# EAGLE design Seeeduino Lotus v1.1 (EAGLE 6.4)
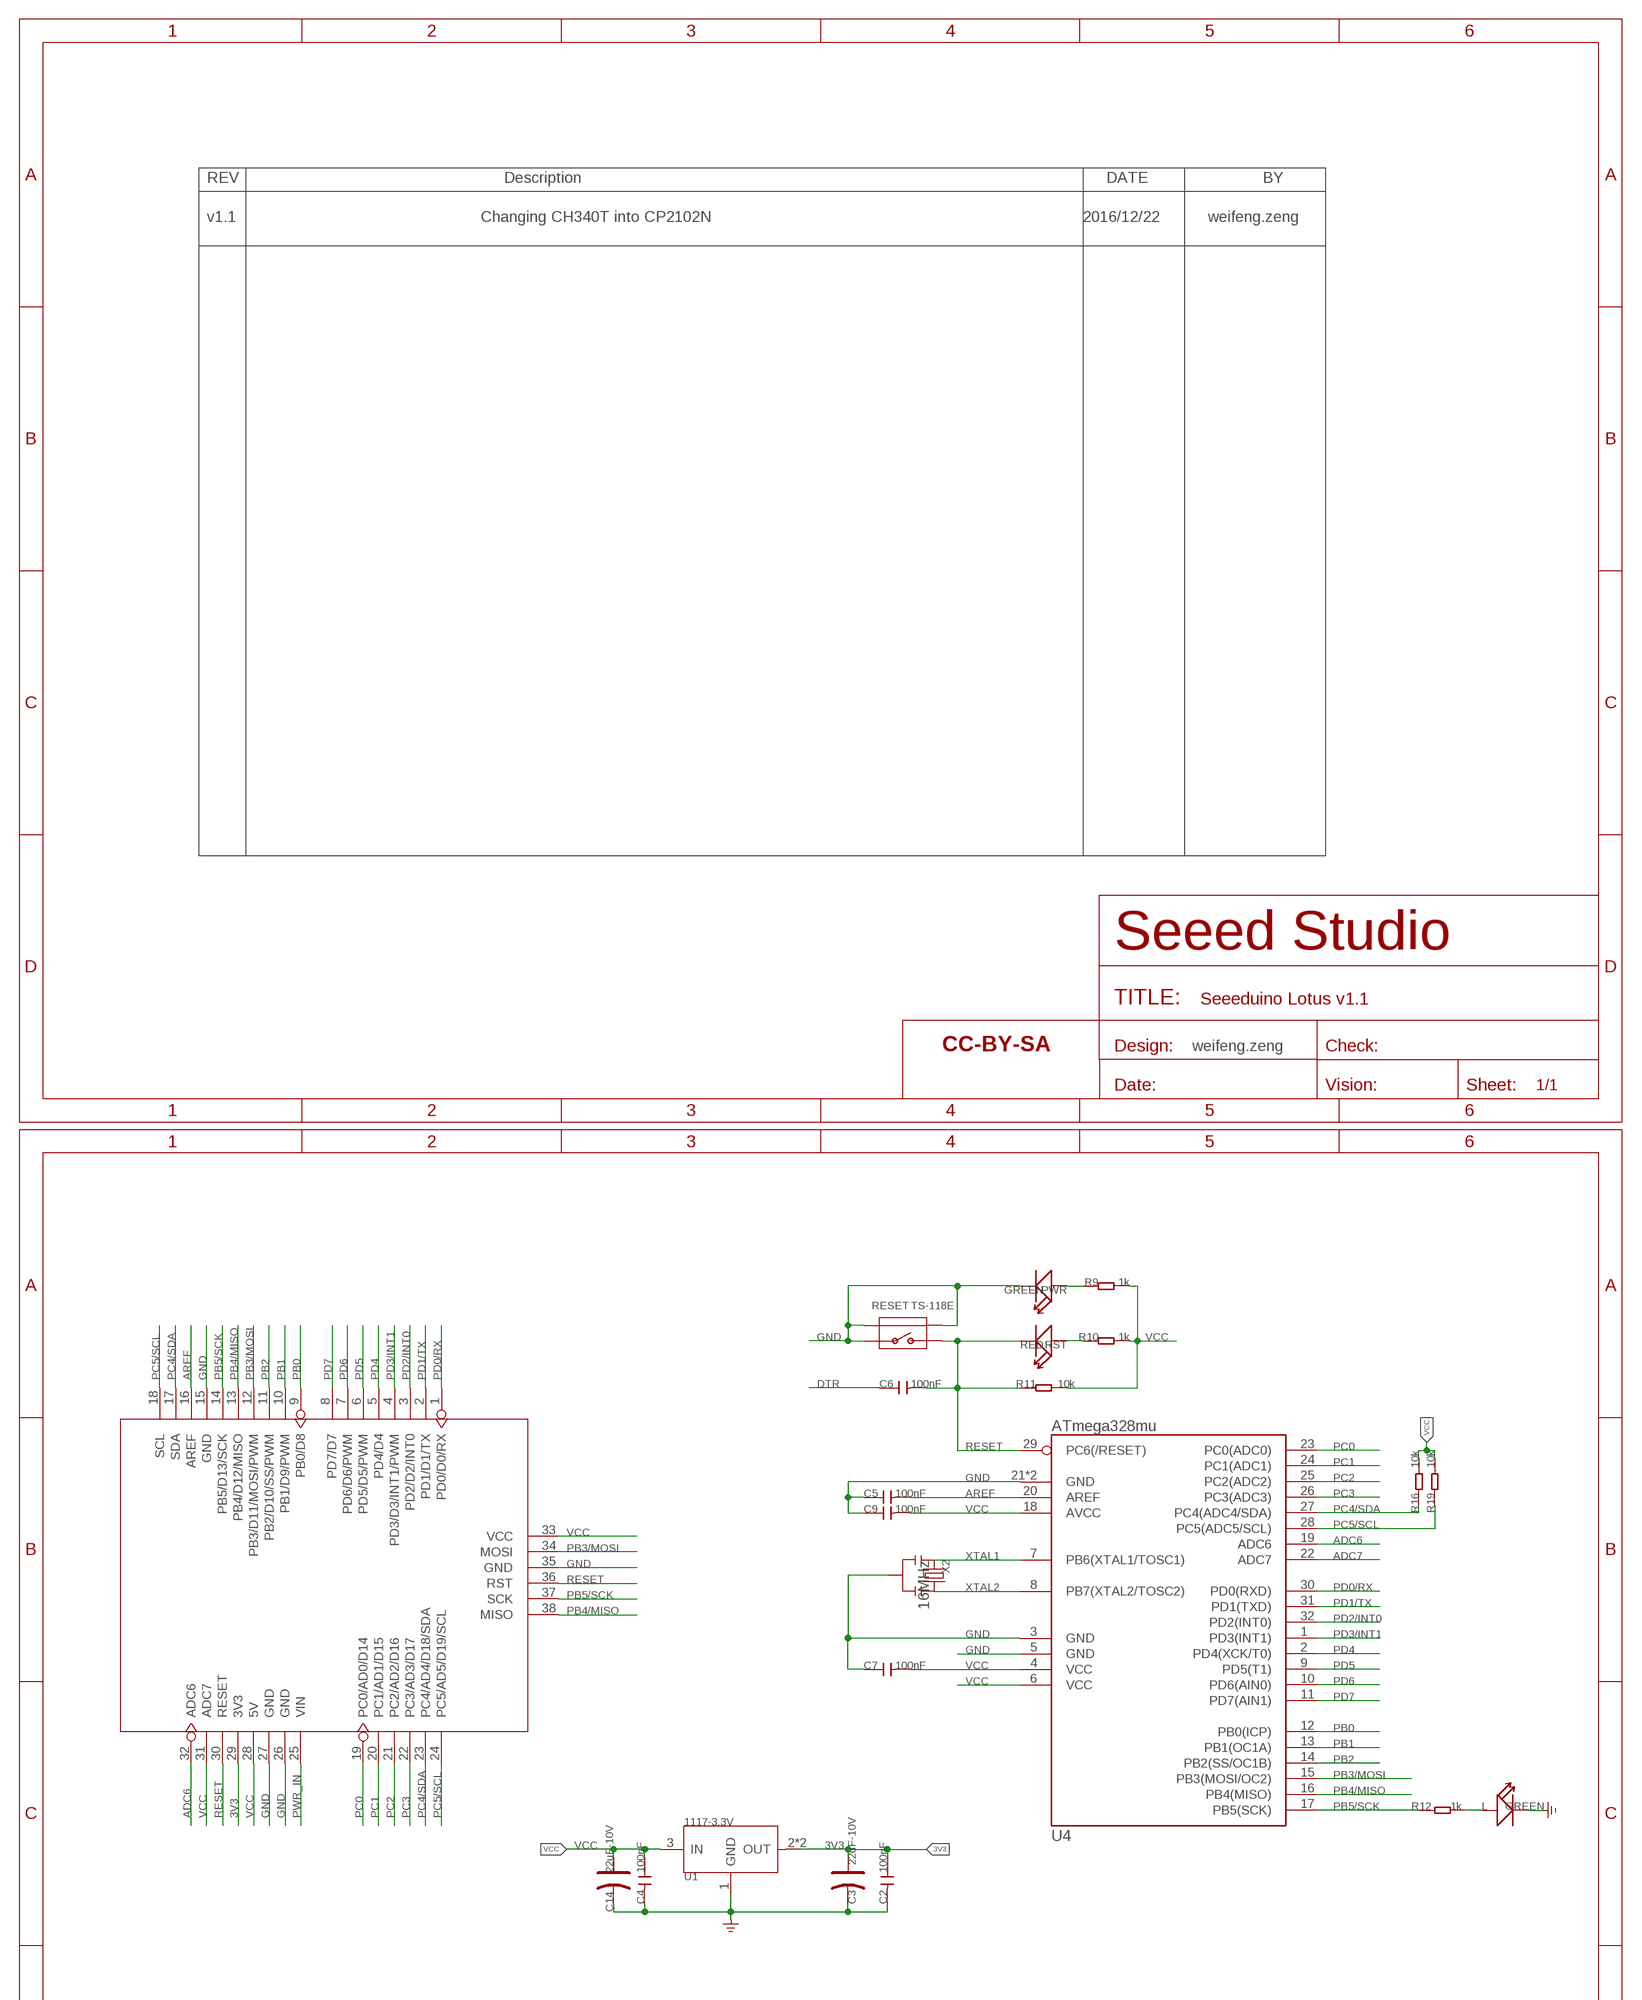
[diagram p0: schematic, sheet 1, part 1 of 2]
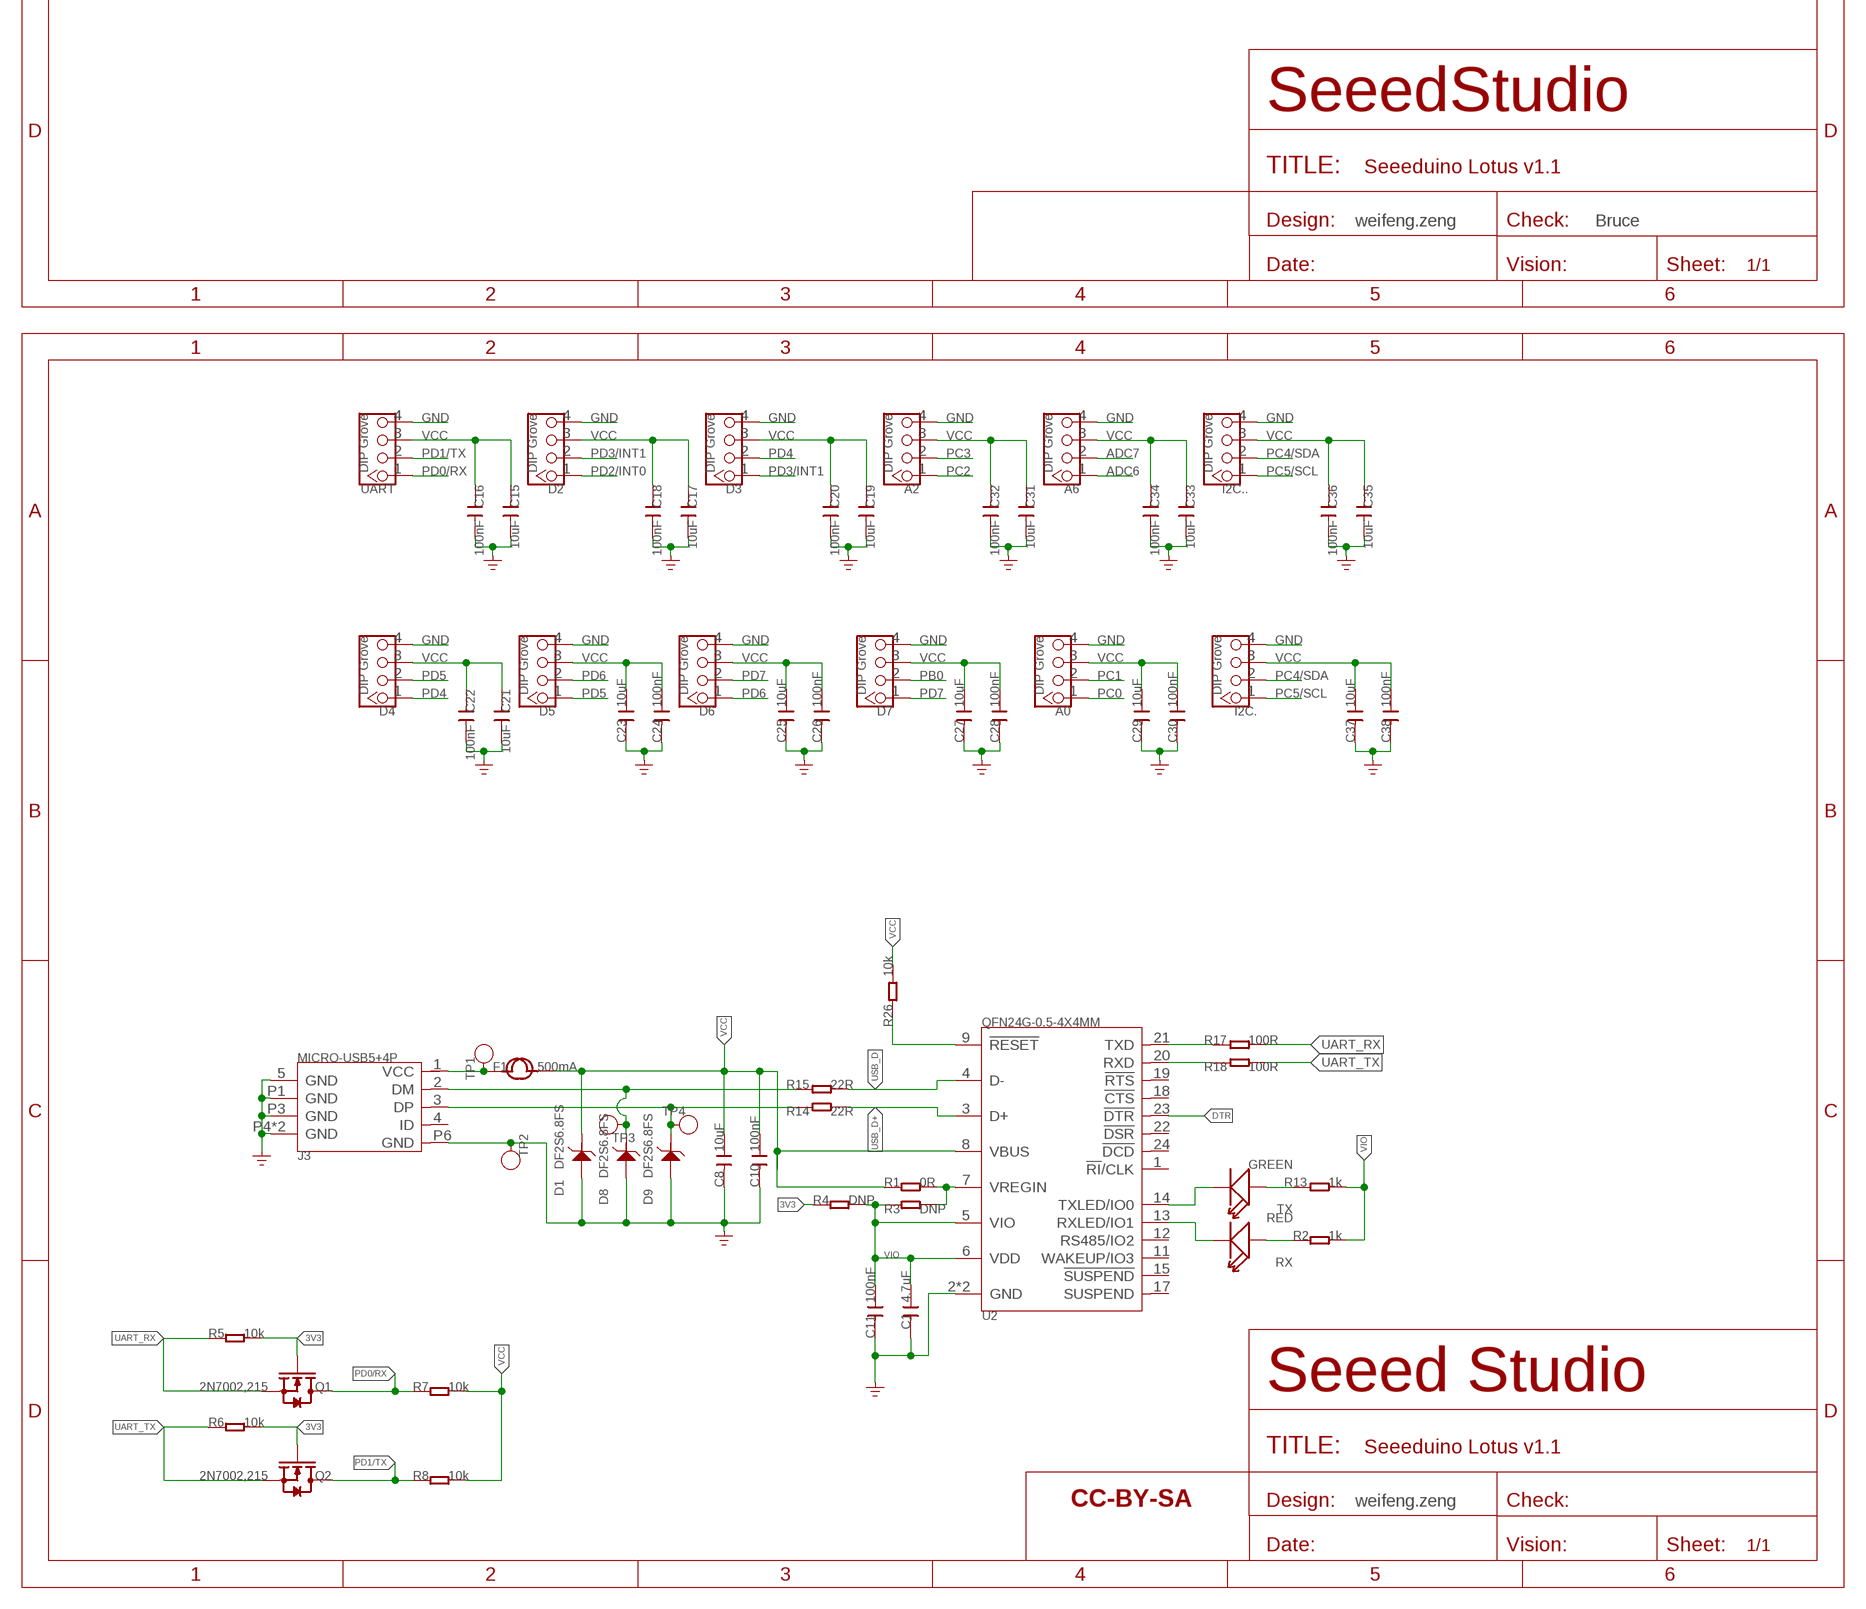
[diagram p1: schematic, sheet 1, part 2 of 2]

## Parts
A0  DIP Grove  TWIG-4P-2.0-2.0  [4P-2.0]
A2  DIP Grove  TWIG-4P-2.0-2.0  [4P-2.0]
A6  DIP Grove  TWIG-4P-2.0-2.0  [4P-2.0]
C1  4.7uF  CAP-0603  [C0603]
C2  100nF  CAP-0603  [C0603]
C3  22uF-10V  CAP-AVX-A  [AVX-A]
C4  100nF  CAP-0603  [C0603]
C5  100nF  CAP-0603  [C0603]
C6  100nF  CAP-0603  [C0603]
C7  100nF  CAP-0603  [C0603]
C8  10uF  CAP-0603  [C0603]
C9  100nF  CAP-0603  [C0603]
C10  100nF  CAP-0603  [C0603]
C11  100nF  CAP-0603  [C0603]
C14  22uF-10V  CAP-AVX-A  [AVX-A]
C15  10uF  CAP-0603  [C0603]
C16  100nF  CAP-0603  [C0603]
C17  10uF  CAP-0603  [C0603]
C18  100nF  CAP-0603  [C0603]
C19  10uF  CAP-0603  [C0603]
C20  100nF  CAP-0603  [C0603]
C21  10uF  CAP-0603  [C0603]
C22  100nF  CAP-0603  [C0603]
C23  10uF  CAP-0603  [C0603]
C24  100nF  CAP-0603  [C0603]
C25  10uF  CAP-0603  [C0603]
C26  100nF  CAP-0603  [C0603]
C27  10uF  CAP-0603  [C0603]
C28  100nF  CAP-0603  [C0603]
C29  10uF  CAP-0603  [C0603]
C30  100nF  CAP-0603  [C0603]
C31  10uF  CAP-0603  [C0603]
C32  100nF  CAP-0603  [C0603]
C33  10uF  CAP-0603  [C0603]
C34  100nF  CAP-0603  [C0603]
C35  10uF  CAP-0603  [C0603]
C36  100nF  CAP-0603  [C0603]
C37  10uF  CAP-0603  [C0603]
C38  100nF  CAP-0603  [C0603]
D1  DF2S6.8FS  D-ESD-2P'DF2S6.8FS'  [SOD-923]
D2  DIP Grove  TWIG-4P-2.0-2.0  [4P-2.0]
D3  DIP Grove  TWIG-4P-2.0-2.0  [4P-2.0]
D4  DIP Grove  TWIG-4P-2.0-2.0  [4P-2.0]
D5  DIP Grove  TWIG-4P-2.0-2.0  [4P-2.0]
D6  DIP Grove  TWIG-4P-2.0-2.0  [4P-2.0]
D7  DIP Grove  TWIG-4P-2.0-2.0  [4P-2.0]
D8  DF2S6.8FS  D-ESD-2P'DF2S6.8FS'  [SOD-923]
D9  DF2S6.8FS  D-ESD-2P'DF2S6.8FS'  [SOD-923]
F1  500mA  FUSE'1206'  [F1206]
FR1  SEEEDSTUDIO-OPEN-SCH-FRAME  [SEEEDSTUDIO-PCB-FRAME]
FR2  SEEEDSTUDIO-OPEN-SCH-FRAME  [SEEEDSTUDIO-PCB-FRAME]
I2C.  DIP Grove  TWIG-4P-2.0-2.0  [4P-2.0]
I2C..  DIP Grove  TWIG-4P-2.0-2.0  [4P-2.0]
J3  MICRO-USB5+4P  [MICRO-USB5+5P-SMD-0.65-7.2X5.06MM]
L  GREEN  LED'0603'  [LED-0603]
PWR  GREEN  LED'0603'  [LED-0603]
Q1  2N7002,215  MOSFET-N'SOT23'  [SOT-23]
Q2  2N7002,215  MOSFET-N'SOT23'  [SOT-23]
R1  0R  RES-0603  [R0603]
R2  1k  RES-0603  [R0603]
R3  DNP  RES-0603  [R0603]
R4  DNP  RES-0603  [R0603]
R5  10k  RES-0603  [R0603]
R6  10k  RES-0603  [R0603]
R7  10k  RES-0603  [R0603]
R8  10k  RES-0603  [R0603]
R9  1k  RES-0603  [R0603]
R10  1k  RES-0603  [R0603]
R11  10k  RES-0603  [R0603]
R12  1k  RES-0603  [R0603]
R13  1k  RES-0603  [R0603]
R14  22R  RES-0603  [R0603]
R15  22R  RES-0603  [R0603]
R16  10k  RES-0603  [R0603]
R17  100R  RES-0603  [R0603]
R18  100R  RES-0603  [R0603]
R19  10k  RES-0603  [R0603]
R26  10k  RES-0603  [R0603]
RESET  TS-118E  BUTTON-4P-REINFORCE'TS-1188E'  [4P-SMD-7X3.5X3.5H]
RST  RED  LED'0603'  [LED-0603]
RX  RED  LED'0603'  [LED-0603]
TP1  TEST-POINT'4545'  [TP-D45MIL]
TP2  TEST-POINT'4545'  [TP-D45MIL]
TP3  TEST-POINT'4545'  [TP-D45MIL]
TP4  TEST-POINT'4545'  [TP-D45MIL]
TX  GREEN  LED'0603'  [LED-0603]
U1  1117-3.3V  LD1117'SOT89'  [SOT89]
U2  QFN24G-0.5-4X4MM  CONVERTER-CP2102N(QFN24)  [QFN24G-0.5-4X4MM]
U3  ARDUINO-38P  [ARDUINO-38P]
U4  ATmega328mu  ATMEGA8/168/328MLF  [MLF32X-W/HEAT]
UART  DIP Grove  TWIG-4P-2.0-2.0  [4P-2.0]
X2  16MHz  CRYSTAL-RESONATOR'SMD'  [RESONATOR3-SMD-3.6X1.3X0.8MM]

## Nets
3V3: C2.1 C3.+ Q1.1(G) Q2.1(G) R4.1 R5.2 R6.2 U1.2(OUT) U1.4(OUT) U3.29(3V3)
ADC6: A6.1 U3.32(ADC6) U4.19(ADC6)
ADC7: A6.2 U4.22(ADC7)
AREF: C5.2 U3.16(AREF) U4.20(AREF)
D-: D8.1 J3.2(DM) R15.1 TP3.T
DTR: C6.1 U2.23(!DTR!)
GND: A0.4 A2.4 A6.4 C1.2 C2.2 C3.- C4.2 C5.1 C7.1 C8.2 C9.1 C10.2 C11.2 C14.- C15.1 C16.1 C17.1 C18.1 C19.1 C20.1 C21.1 C22.1 C23.2 C24.2 C25.2 C26.2 C27.2 C28.2 C29.2 C30.2 C31.1 C32.1 C33.1 C34.1 C35.1 C36.1 C37.2 C38.2 D1.2 D2.4 D3.4 D4.4 D5.4 D6.4 D7.4 D8.2 D9.2 I2C..4 I2C...4 J3.5(GND) J3.P1(GND) J3.P3(GND) J3.P4(GND) J3.P5(GND) J3.P6(GND) L.- PWR.- RESET.1 RESET.S1 RESET.S2 TP2.T U1.1(GND) U2.2(GND) U2.PAD(GND) U3.15(GND) U3.26(GND) U3.27(GND) U3.35(GND) U4.3(GND) U4.5(GND) U4.21(GND) U4.HEAT(GND) UART.4 X2.2 ; supply symbol labelled GND_POWER
N$1: R1.2 R3.2 U2.7(VREGIN)
N$2: R10.2 RST.+
N$3: PWR.+ R9.2
N$4: R26.2 U2.9(!RESET!)
N$5: TX.- U2.14(TXLED/IO0)
N$7: F1.1 J3.1(VCC) TP1.T
N$10: RX.- U2.13(RXLED/IO1)
N$11: D9.1 J3.3(DP) R14.1 TP4.T
N$13: L.+ R12.2
N$17: R18.1 U2.20(RXD)
N$18: R17.1 U2.21(TXD)
N$36: R2.1 RX.+
N$37: R13.1 TX.+
PB0: D7.2 U3.9(PB0/D8) U4.12(PB0(ICP))
PB1: U3.10(PB1/D9/PWM) U4.13(PB1(OC1A))
PB2: U3.11(PB2/D10/SS/PWM) U4.14(PB2(SS/OC1B))
PB3/MOSI: U3.12(PB3/D11/MOSI/PWM) U3.34(MOSI) U4.15(PB3(MOSI/OC2))
PB4/MISO: U3.13(PB4/D12/MISO) U3.38(MISO) U4.16(PB4(MISO))
PB5/SCK: R12.1 U3.14(PB5/D13/SCK) U3.37(SCK) U4.17(PB5(SCK))
PC0: A0.1 U3.19(PC0/AD0/D14) U4.23(PC0(ADC0))
PC1: A0.2 U3.20(PC1/AD1/D15) U4.24(PC1(ADC1))
PC2: A2.1 U3.21(PC2/AD2/D16) U4.25(PC2(ADC2))
PC3: A2.2 U3.22(PC3/AD3/D17) U4.26(PC3(ADC3))
PC4/SDA: I2C..2 I2C...2 R16.2 U3.17(SDA) U3.23(PC4/AD4/D18/SDA) U4.27(PC4(ADC4/SDA))
PC5/SCL: I2C..1 I2C...1 R19.2 U3.18(SCL) U3.24(PC5/AD5/D19/SCL) U4.28(PC5(ADC5/SCL))
PD0/RX: Q1.3(D) R7.1 U3.1(PD0/D0/RX) U4.30(PD0(RXD)) UART.1
PD1/TX: Q2.3(D) R8.1 U3.2(PD1/D1/TX) U4.31(PD1(TXD)) UART.2
PD2/INT0: D2.1 U3.3(PD2/D2/INT0) U4.32(PD2(INT0))
PD3/INT1: D2.2 D3.1 U3.4(PD3/D3/INT1/PWM) U4.1(PD3(INT1))
PD4: D3.2 D4.1 U3.5(PD4/D4) U4.2(PD4(XCK/T0))
PD5: D4.2 D5.1 U3.6(PD5/D5/PWM) U4.9(PD5(T1))
PD6: D5.2 D6.1 U3.7(PD6/D6/PWM) U4.10(PD6(AIN0))
PD7: D6.2 D7.1 U3.8(PD7/D7) U4.11(PD7(AIN1))
PWR_IN: U3.25(VIN)
RESET: C6.2 R11.2 RESET.2 RST.- U3.30(RESET) U3.36(RST) U4.29(PC6(/RESET))
UART_RX: Q1.2(S) R5.1 R17.2
UART_TX: Q2.2(S) R6.1 R18.2
USB_D: R15.2 U2.4(D-)
USB_D+: R14.2 U2.3(D+)
VCC: A0.3 A2.3 A6.3 C4.1 C7.2 C8.1 C9.2 C10.1 C14.+ C15.2 C16.2 C17.2 C18.2 C19.2 C20.2 C21.2 C22.2 C23.1 C24.1 C25.1 C26.1 C27.1 C28.1 C29.1 C30.1 C31.2 C32.2 C33.2 C34.2 C35.2 C36.2 C37.1 C38.1 D1.1 D2.3 D3.3 D4.3 D5.3 D6.3 D7.3 F1.2 I2C..3 I2C...3 R1.1 R7.2 R8.2 R9.1 R10.1 R11.1 R16.1 R19.1 R26.1 U1.3(IN) U2.8(VBUS) U3.28(5V) U3.31(ADC7) U3.33(VCC) U4.4(VCC) U4.6(VCC) U4.18(AVCC) UART.3
VIO: C1.1 C11.1 R2.2 R3.1 R4.2 R13.2 U2.5(VIO) U2.6(VDD)
XTAL1: U4.7(PB6(XTAL1/TOSC1)) X2.1
XTAL2: U4.8(PB7(XTAL2/TOSC2)) X2.3
Unconnected: J3.4(ID) U2.1(!RI!/CLK) U2.11(WAKEUP/IO3) U2.12(RS485/IO2) U2.15(!SUSPEND!) U2.17(SUSPEND) U2.18(!CTS!) U2.19(!RTS!) U2.22(!DSR!) U2.24(!DCD!)

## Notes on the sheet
- v1.1 | Changing CH340T into CP2102N | 2016/12/22 | weifeng.zeng
- weifeng.zeng
- weifeng.zeng | Bruce
- weifeng.zeng

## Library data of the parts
A0 A2 A6 = Connector :TWIG-4P-2.0
C1 C2 C4 C8 C10 C11 C15-C38 = Discrete-new:CAP: Ceramic Capacitors
C3 C14 = Discrete:CAP*: Electrolytic Capacitors,Tantalum Capacitors and Super Capacitors
C5-C7 C9 = C-R-package test:CAP: Ceramic Capacitors
D1 D8 D9 = Discrete-new:D-ESD-2P: SOD-923:304060009;SOD-123:304060001
D2-D7 I2C. I2C.. UART = Connector:TWIG-4P-2.0
F1 = Discrete-new:FUSE
FR1 FR2 = moudle-new:SEEEDSTUDIO-OPEN-SCH-FRAME
J3 = Connector-new:MICRO-USB5+4P: 5+4P-SMD-0.65-B:320010000;5+2P-SMD-0.65-AB:340032001;5+5P-SMD-0.65-7.2X5.06MM:320010050;
L PWR RST = Discrete:LED*
Q1 Q2 = Discrete-new:MOSFET-N
R1-R8 R13-R19 R26 = Discrete-new:RES
R9-R12 = C-R-package test:RES
RESET = Discrete:BUTTON-4P-REINFORCE: TS-1188E http://www.best-dz.com/?thread-374-2.html
RX TX = Discrete-new:LED
TP1-TP4 = Discrete-new:TEST-POINT; PARTNO: DNP
U1 = IC:LD1117: Low Drop Fixed And Adjustable Positive Voltage Regulators http://www.datasheetcatalog.org/datasheet/SGSThomsonMicroelectronics/mXuqtqv.pdf
U2 = template:CONVERTER-CP2102N(QFN24)
U3 = moudle:ARDUINO-38P
U4 = IC:ATMEGA8/168/328: MICROCONTROLLER
X2 = Discrete-new:CRYSTAL-RESONATOR: Resonator Small SMD resonator. This is the itty bitty 10/20MHz resonators with built in caps. CSTCE10M0G55 and CSTCE20M0V53. Footprint has been reviewed closely but hasn't been tested yet.

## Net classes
3 usbvcc: width 0.203 mm, drill 0.305 mm, clearance 0.203 mm

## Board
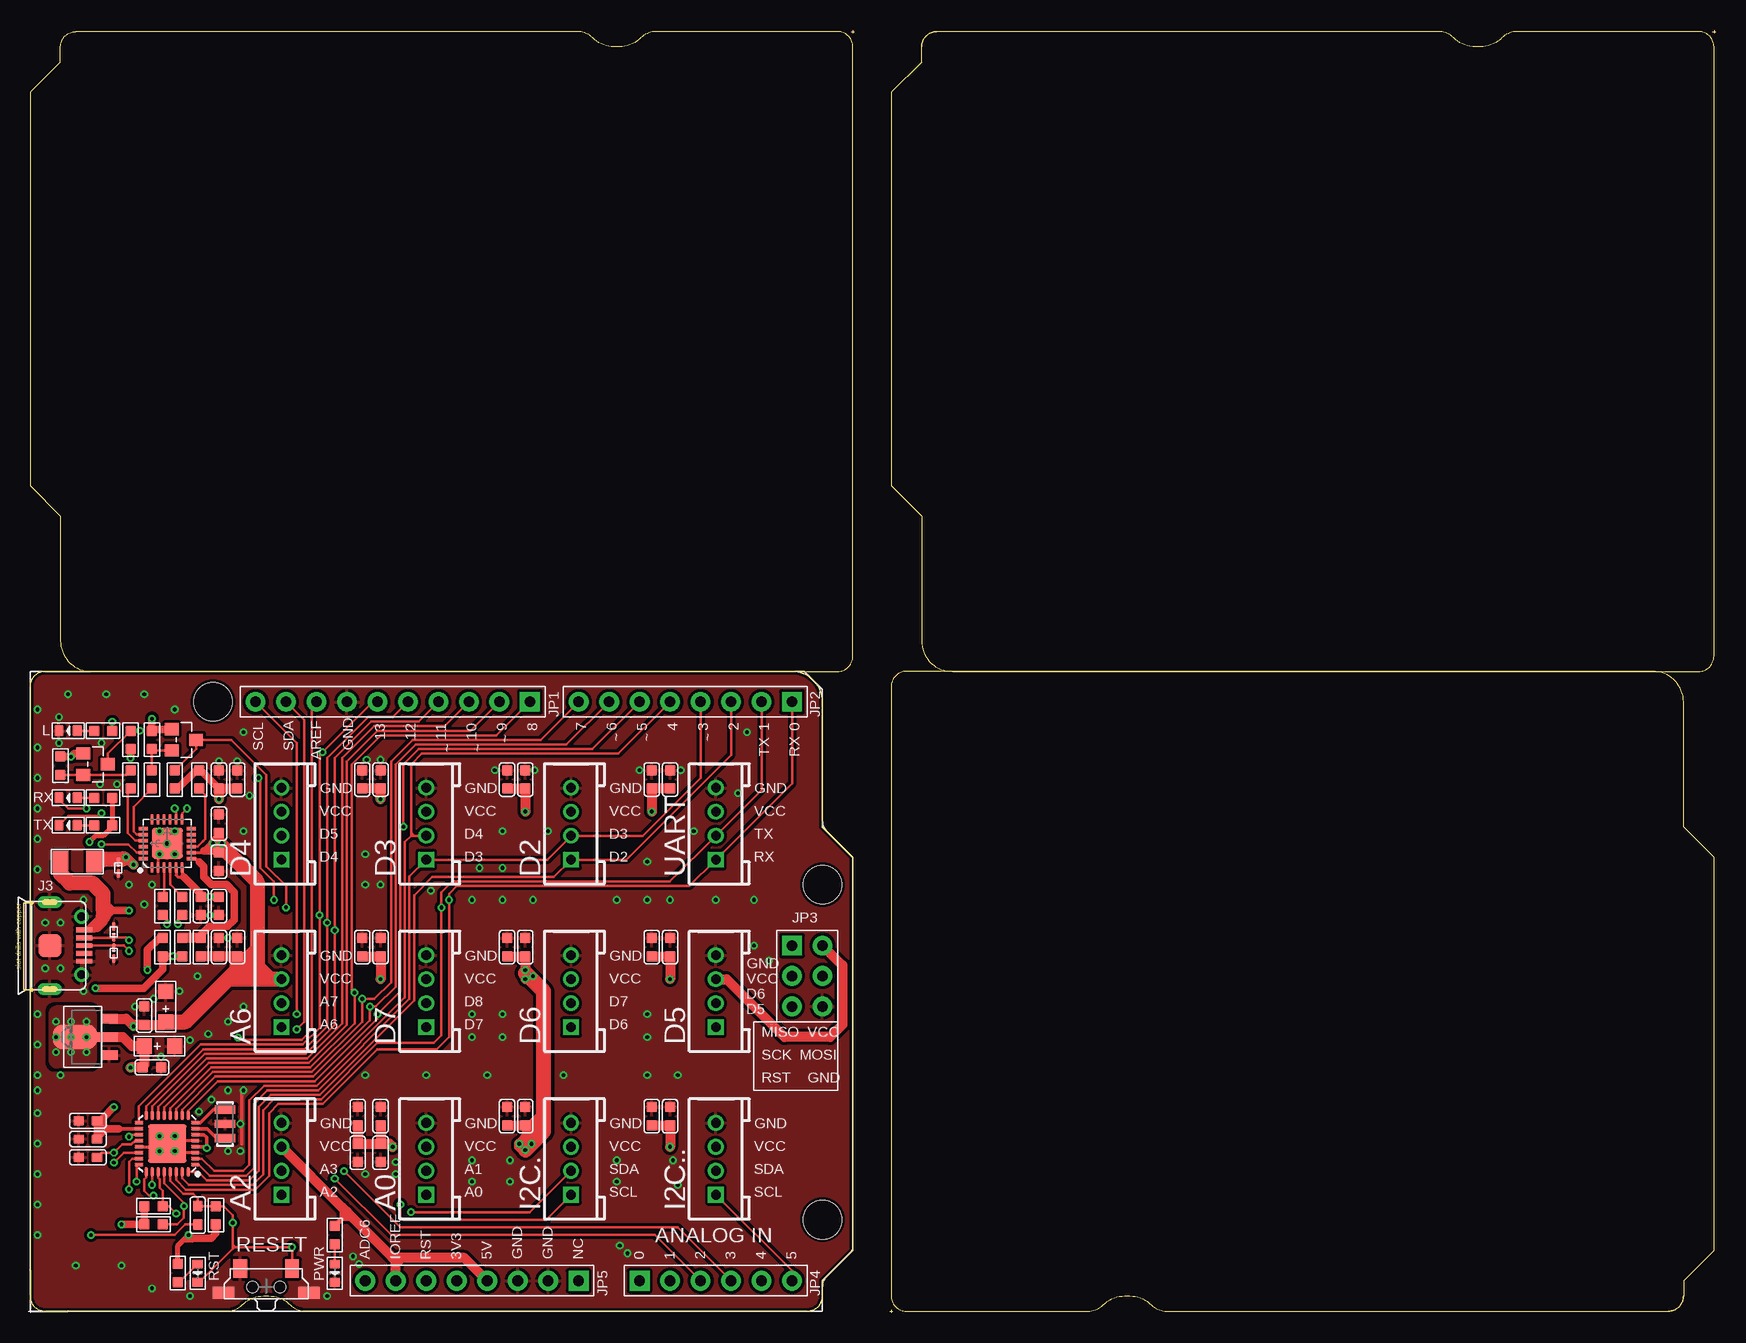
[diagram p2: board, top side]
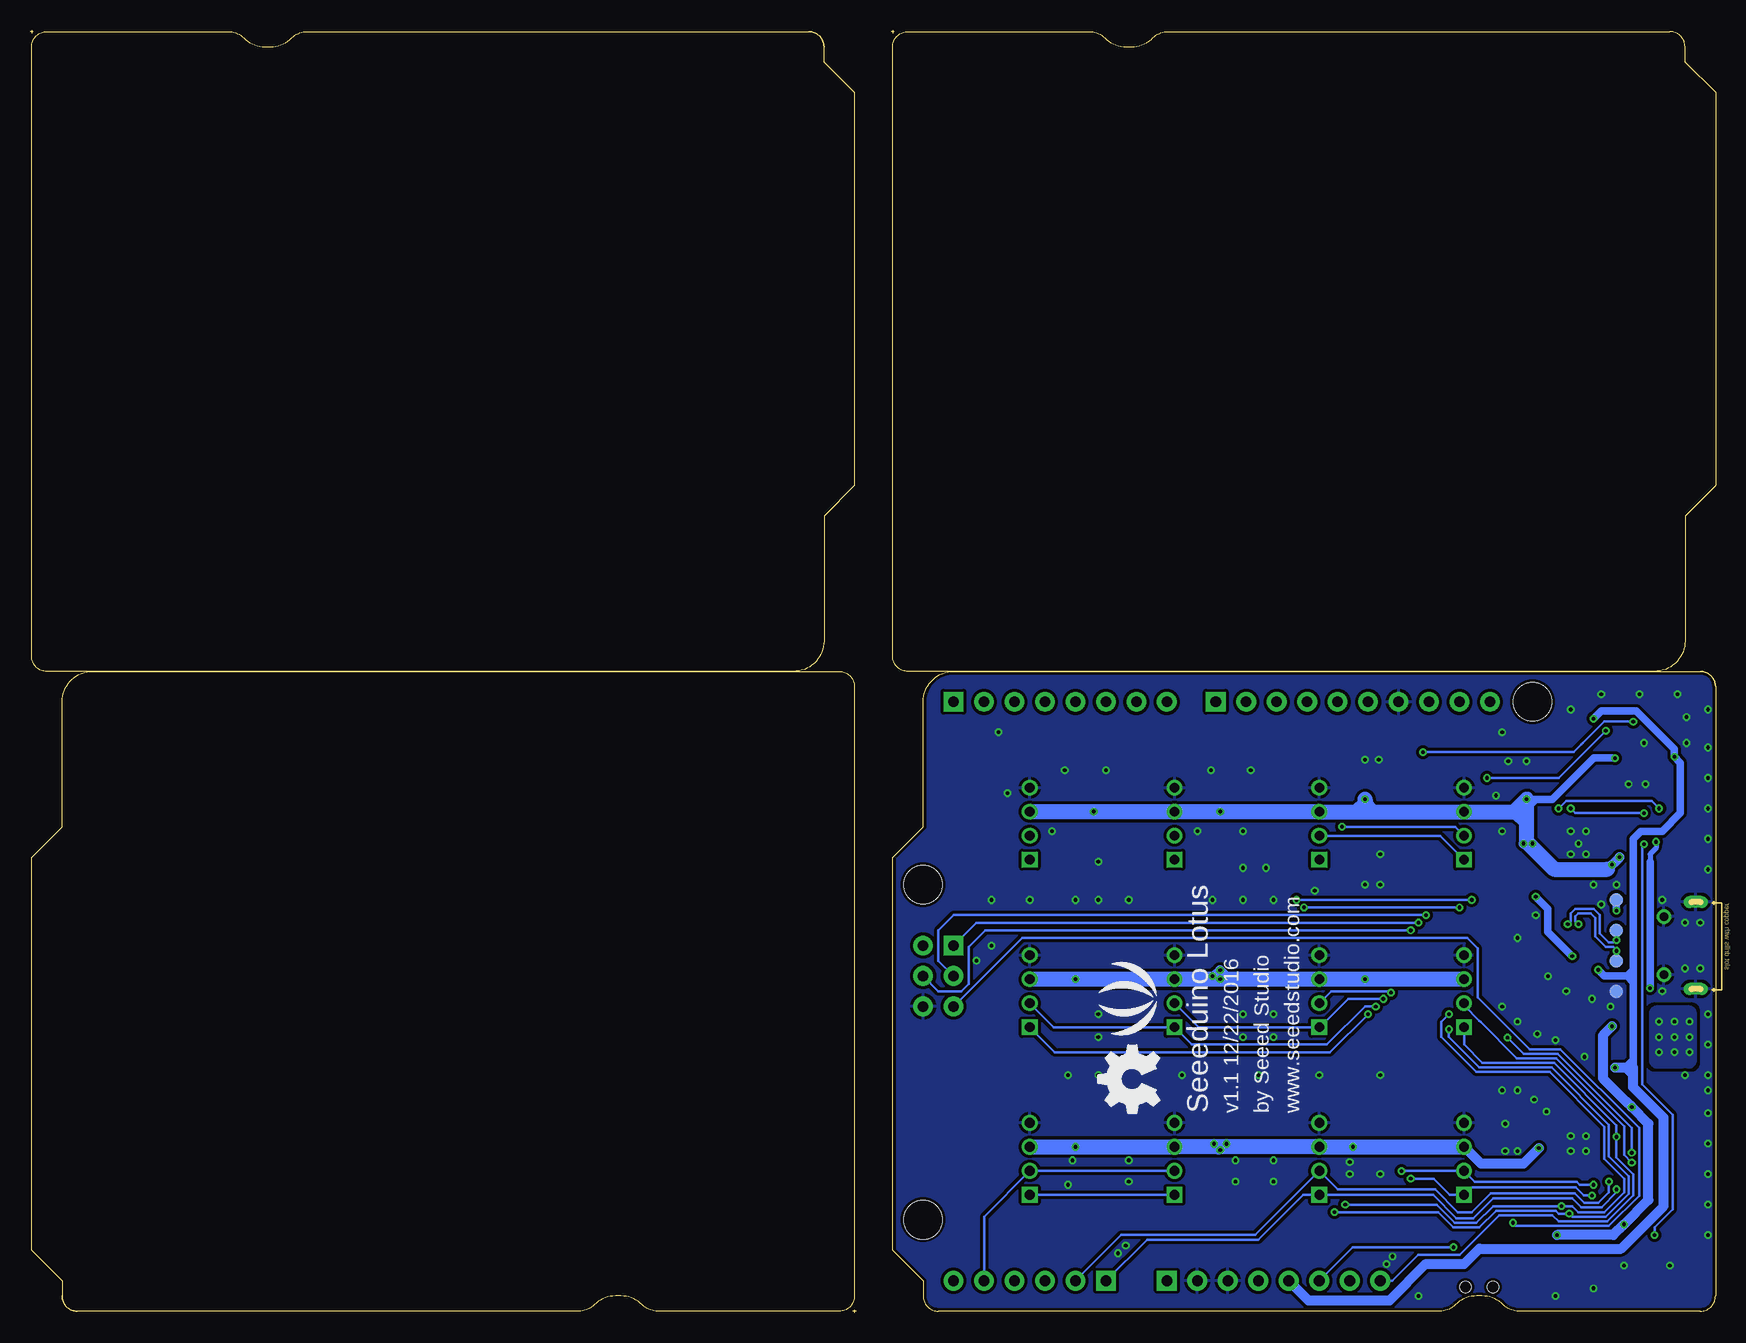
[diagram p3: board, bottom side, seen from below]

Size 140.46 x 106.93 mm. Coordinates in mm from the lower left corner, seen from the top.
Outline: 125 segments
Copper layers (1*16): Top 0.035mm / dielectric 1.5mm / Bottom 0.035mm
Design rules "SeeedStudio_rule_no_angle_090911 *": minimum track width 1mil, minimum drill 12mil, track to track 6mil, track to pad 6mil, pad to pad 6mil, via to via 6mil, smd to smd 0mil, copper to edge 10mil, drill to drill 10mil, minimum pad ring 10mil, minimum via ring 6mil, stop-mask expansion 2mil, vias tented up to drill 100mil, thermal gap 10mil
Holes 2.03 mm at 7.62,111.25 132.72,111.25 132.72,-4.32 7.62,-4.32

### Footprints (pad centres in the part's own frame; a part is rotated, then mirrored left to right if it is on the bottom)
4P-2.0 = drill 0.8 pad 1.27 square: 1 -3,0 | drill 0.8 pad 1.27: 2 -1,0; 3 1,0; 4 3,0
C0603 = smd 0.889 x 0.889: 1 0,0.762; 2 0,-0.762
AVX-A = smd 1.27 x 1.27: + -1.27,0; - 1.27,0
C0603' = smd 0.762 x 0.889: 1 0,0.762; 2 0,-0.762
SOD-923 = smd 0.7 x 0.3: 1 -0.45,0; 2 0.45,0
F1206 = smd 1.27 x 1.778: 1 -1.397,0; 2 1.397,0
MICRO-USB5+5P-SMD-0.65-7.2X5.06MM = smd 0.4 x 1.35: 1 -1.3,2.875; 2 -0.65,2.875; 3 0,2.875; 4 0.65,2.875; 5 1.3,2.875 | smd 1.9 x 1.9: P1 0,0 | drill 0.508 pad 1.016 long: P3 -3.625,0; P4 3.625,0 | drill 0.7: P5 -2.425,2.65; P6 2.425,2.65
LED-0603 = smd 0.762 x 0.889: + -0.762,0; - 0.762,0
SOT-23 = smd 1.016 x 1.143: 1 -0.889,-1.016; 2 0.889,-1.016; 3 0,1.016
R0603 = smd 0.889 x 0.889: 1 0,0.762; 2 0,-0.762
4P-SMD-7X3.5X3.5H = smd 1.143 x 1.524: 1 -2.159,1.524; 2 2.159,1.524 | smd 1.778 x 1.016: S1 -3.556,-0.508; S2 3.556,-0.508 | hole 0.95: -1.15,0; 1.15,0
TP-D45MIL = smd 1.143 x 1.143: T 0,0
SOT89 = smd 0.8 x 1.4: 1 -1.524,-1.905; 3 1.524,-1.905 | smd 0.8 x 1.9: 2 0,-1.651 | smd 2.032 x 3.65: 4 0,0.94
QFN24G-0.5-4X4MM = smd 0.8 x 0.26: 1 -2,1.25; 2 -2,0.75; 3 -2,0.25; 4 -2,-0.25; 5 -2,-0.75; 6 -2,-1.25; 13 2,-1.25; 14 2,-0.75; 15 2,-0.25; 16 2,0.25; 17 2,0.75; 18 2,1.25 | smd 0.26 x 0.8: 7 -1.25,-2; 8 -0.75,-2; 9 -0.25,-2; 10 0.25,-2; 11 0.75,-2; 12 1.25,-2; 19 1.25,2; 20 0.75,2; 21 0.25,2; 22 -0.25,2; 23 -0.75,2; 24 -1.25,2 | smd 2.6 x 2.6: PAD 0.02,-0.01
ARDUINO-38P = drill 0.889 pad 1.651 square: 1 63.5,50.8; 9 41.656,50.8; 19 50.8,2.54; 25 45.72,2.54; 38 63.5,30.48 | drill 0.889 pad 1.651: 2 60.96,50.8; 3 58.42,50.8; 4 55.88,50.8; 5 53.34,50.8; 6 50.8,50.8; 7 48.26,50.8; 8 45.72,50.8; 10 39.116,50.8; 11 36.576,50.8; 12 34.036,50.8; 13 31.496,50.8; 14 28.956,50.8; 15 26.416,50.8; 16 23.876,50.8; 17 21.336,50.8; 18 18.796,50.8; 20 53.34,2.54; 21 55.88,2.54; 22 58.42,2.54; 23 60.96,2.54; 24 63.5,2.54; 26 43.18,2.54; 27 40.64,2.54; 28 38.1,2.54; 29 35.56,2.54; 30 33.02,2.54; 31 30.48,2.54; 32 27.94,2.54; 33 66.04,30.48; 34 66.04,27.94; 35 66.04,25.4; 36 63.5,25.4; 37 63.5,27.94 | hole 3.2: 15.24,50.8; 66.04,35.56; 66.04,7.62
MLF32X-W/HEAT = smd 0.7 x 0.3: 1 -2.35,1.75; 2 -2.35,1.25; 3 -2.35,0.75; 4 -2.35,0.25; 5 -2.35,-0.25; 6 -2.35,-0.75; 7 -2.35,-1.25; 8 -2.35,-1.75; 17 2.35,-1.75; 18 2.35,-1.25; 19 2.35,-0.75; 20 2.35,-0.25; 21 2.35,0.25; 22 2.35,0.75; 23 2.35,1.25; 24 2.35,1.75 | smd 0.3 x 0.7: 9 -1.75,-2.35; 10 -1.25,-2.35; 11 -0.75,-2.35; 12 -0.25,-2.35; 13 0.25,-2.35; 14 0.75,-2.35; 15 1.25,-2.35; 16 1.75,-2.35; 25 1.75,2.35; 26 1.25,2.35; 27 0.75,2.35; 28 0.25,2.35; 29 -0.25,2.35; 30 -0.75,2.35; 31 -1.25,2.35; 32 -1.75,2.35 | smd 3.175 x 3.175: HEAT 0,0
RESONATOR3-SMD-3.6X1.3X0.8MM = smd 0.7 x 1.7: 1 -1.2,0; 2 0,0; 3 1.2,0

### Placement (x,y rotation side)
A0  33.02,12.83 90 top
A2  20.95,12.83 90 top
A6  20.95,26.8 90 top
C1  15.75,33.91 0 top
C2  10.16,20.45 90 top
C3  10.79,22.22 0 top
C4  9.53,24.77 180 top
C5  100nF  [C0603']  4.83,12.95 90 top
C6  100nF  [C0603']  13.97,8.13 180 top
C7  100nF  [C0603']  4.83,16 90 top
C8  15.75,37.59 0 top
C9  100nF  [C0603']  4.83,14.48 90 top
C10  15.75,40.77 180 top
C11  14.22,33.91 0 top
C14  11.3,25.53 90 top
C15  51.82,44.45 0 top
C16  53.34,44.45 0 top
C17  39.75,44.45 0 top
C18  41.27,44.45 0 top
C19  27.69,44.45 0 top
C20  29.21,44.45 0 top
C21  15.75,44.45 0 top
C22  17.27,44.45 0 top
C23  51.82,30.48 180 top
C24  53.34,30.48 180 top
C25  39.75,30.48 180 top
C26  41.27,30.48 180 top
C27  27.69,30.48 180 top
C28  29.21,30.48 180 top
C29  29.21,13.34 0 top
C30  29.21,16.38 180 top
C31  27.3,13.34 180 top
C32  27.3,16.38 0 top
C33  15.75,30.48 0 top
C34  17.27,30.48 0 top
C35  51.82,16.38 0 top
C36  53.34,16.38 0 top
C37  39.75,16.38 180 top
C38  41.27,16.38 180 top
D1  7.37,37.08 270 top
D2  45.09,40.77 90 top
D3  33.02,40.77 90 top
D4  20.95,40.77 90 top
D5  57.15,26.8 90 top
D6  45.09,26.8 90 top
D7  33.02,26.8 90 top
D8  6.99,31.75 90 top
D9  6.99,29.97 270 top
F1  3.94,37.59 0 top
FR1  not placed on the board
FR2  not placed on the board
I2C.  45.09,12.83 90 top
I2C..  57.15,12.83 90 top
J3  1.65,30.61 270 top
L  3.17,48.51 180 top
PWR  25.4,3.3 270 top
Q1  5.46,45.72 270 top
Q2  12.83,47.75 270 top
R1  14.22,30.48 180 top
R2  6.1,42.93 90 top
R3  12.7,30.48 180 top
R4  11.05,30.48 0 top
R5  2.54,45.59 180 top
R6  10.16,47.75 180 top
R7  8.38,47.75 0 top
R8  12.06,44.45 0 top
R9  25.4,6.48 0 top
R10  12.32,3.3 0 top
R11  15.49,8.13 180 top
R12  6.1,48.51 270 top
R13  6.1,40.64 90 top
R14  11.05,33.91 180 top
R15  12.7,33.91 180 top
R16  10.29,8.89 90 top
R17  8.38,44.45 180 top
R18  10.16,44.45 180 top
R19  10.29,7.37 90 top
R26  14.1,44.45 0 top
RESET  19.68,2.16 0 top
RST  13.97,3.3 270 top
RX  3.17,42.93 180 top
TP1  8.26,34.42 180 bottom
TP2  8.26,26.8 180 bottom
TP3  8.26,31.88 180 bottom
TP4  8.26,29.34 180 bottom
TX  3.17,40.64 180 top
U1  4.7,22.99 90 top
U2  11.43,39.12 90 top
U3  0,0.13 0 top
U4  11.43,14.1 180 top
U$2  [OSHW_FILLX200_NOTEXT]  46.35,16.64 90 bottom
U$4  [LOGO_SILK]  48.26,26.16 90 bottom
U$12  [SEEED_MASK]  3.81,2.67 0 top
UART  57.15,40.77 90 top
X2  16.26,15.75 90 top

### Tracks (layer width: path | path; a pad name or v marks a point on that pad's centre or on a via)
3V3  (via drill 0.3 pad 0.64)
  Top 0.61: v4.7,22.99 U1.4 | 9.53,20.57 C2.1 | R4.1 10.79,31.24 9.78,30.23 v9.78,28.57 | R5.2 v3.43,46.36 3.68,46.61 Q1.1 | Q2.1 10.29,48.64 R6.2 v10.16,49.53
  Top 0.813: C2.1 9.27,20.45 | 9.27,20.45 v8.38,20.45 | 9.27,20.45 9.53,20.7 C3.+ 8.51,22.22 7.75,22.99 U1.2
  Bottom 0.61: 6.86,20.45 6.86,21.08 | 6.86,21.08 6.86,27.56 | 6.86,27.56 6.86,28.07 | 6.86,28.07 6.86,28.57 | 7.37,28.07 6.86,28.07 | 7.37,28.07 6.86,28.57 | 7.37,28.07 6.86,27.56 | 7.37,28.07 9.27,28.07 v9.78,28.57 | 6.86,28.57 6.86,39.5 6.22,40.13 4.45,40.13 2.92,41.66 2.92,45.85 v3.43,46.36 3.43,46.99 6.6,50.16 9.53,50.16 v10.16,49.53 | 6.86,21.08 7.49,20.45 | 7.75,20.45 7.62,20.45 6.86,19.68
  Bottom 0.813: U3.29 33.91,1.02 27.18,1.02 24.13,4.06 20.95,4.06 19.68,5.33 7.87,5.33 4.32,8.89 4.32,16.26 6.86,18.8 6.86,19.68 6.86,20.45 7.49,20.45 7.75,20.45 v8.38,20.45
  other vias: 4.7,24.26 3.43,24.26 2.16,24.26 3.43,22.99 2.16,22.99 2.16,21.72 3.43,21.72 4.7,21.72
  pour Top (isolate 0.254, no thermals): 4.83,20.45 2.29,20.45 arc-90 1.65,21.08 1.65,24.89 arc-90 2.29,25.53 4.83,25.53 arc-90 5.46,24.89 5.46,21.08 arc-90
  pour Bottom (isolate 0.254, no thermals): 4.83,20.45 2.29,20.45 arc-90 1.65,21.08 1.65,24.89 arc-90 2.29,25.53 4.83,25.53 arc-90 5.46,24.89 5.46,21.08 arc-90
ADC6  (via drill 0.3 pad 0.64)
  Top 0.203: U4.19 8.43,14.85 v8.26,14.67
  Bottom 0.203: U3.32 26.92,2.67 24.77,4.83 21.34,4.83 18.03,8.13 13.59,8.13 13.08,7.62 9.02,7.62 6.86,9.78 6.86,11.56 8.26,12.95 v8.26,14.67 8.26,15.63 13.46,20.83 19.43,20.83 20.95,22.35 A6.1
ADC7  (via drill 0.3 pad 0.64)
  Top 0.203: U4.22 7.82,13.35 v6.99,12.51
  Bottom 0.203: v6.99,12.51 7.62,13.15 7.62,15.54 13.28,21.21 16.56,21.21 19.58,24.23 19.68,24.33 20.95,25.6 A6.2
AREF  (via drill 0.3 pad 0.64)
  Top 0.203: U3.16 23.5,50.55 23.5,23.62 22.63,22.75 17.51,22.75 v17.34,22.92 | U4.20 8.76,14.35 8.45,14.03 7.68,14.03 v6.99,13.34 5.97,13.34 C5.2
  Bottom 0.203: v6.99,13.34 6.99,15.43 13.14,21.59 16,21.59 v17.34,22.92
D-  (via drill 0.3 pad 0.64)
  Top 0.203: J3.2 6.94,31.26 D8.1 8.01,31.3 v8.26,31.05 | R15.1 12.32,32.77 v12.32,32.39
  Bottom 0.203: TP3.T v8.26,31.05 8.32,31.05 8.51,30.86 8.89,30.86 9.65,31.62 9.65,33.15 10.16,33.66 11.68,33.66 12.06,33.27 12.06,32.64 v12.32,32.39
DTR  (via drill 0.3 pad 0.64)
  Top 0.203: C6.1 12.95,7.37 12.06,6.48 v5.08,6.48 | U2.23 8.88,38.37 8.19,39.05 v5.97,39.05
  Bottom 0.203: v5.97,39.05 6.1,38.93 6.1,19.05 3.56,16.51 3.56,8.64 5.08,7.11 v5.08,6.48
GND  (via drill 0.3 pad 0.64)
  Top 0.203: U2.2 10.68,38.11 v10.79,38.23
  Top 0.254: U4.21 9.91,13.85 v10.79,14.73 U4.HEAT | U4.3 12.18,13.35 v12.06,13.46 | U4.5 12.45,14.35 v12.06,14.73
  Top 0.305: 17.65,14.1 17.65,18.54
  other vias: 36.83,24.89 39.37,24.89 39.37,22.99 36.83,22.99 51.44,24.89 51.44,22.99 48.9,12.7 40.01,10.92 53.59,12.7 48.9,10.92 40.01,12.7 53.98,10.67 30.48,12.57 26.92,4.7 27.43,4.06 60.33,30.61 61.59,29.34 37.47,37.08 39.37,37.08 49.15,5.59 49.78,4.95 30.48,11.56 36.83,10.92 36.83,12.7 10.79,13.46 0.64,19.81 2.54,19.81 0.64,18.54 0.64,6.48 7.62,3.94 17.78,18.54 17.53,15.75 16.51,13.46 17.53,13.46 27.94,11.56 27.94,19.81 33.02,19.81 38.1,19.81 44.45,19.81 51.44,19.81 53.98,19.81 36.83,34.42 39.37,34.42 41.91,34.42 43.18,40.13 39.37,40.13 51.44,37.59 48.9,34.42 51.44,34.42 53.34,34.42 60.33,34.42 57.15,34.42 3.81,3.94 14.99,33.15 16.51,31.24 29.21,46.1 28.07,46.1 29.21,35.69 27.94,35.69 11.43,39.12 12.06,40.13 10.79,40.13 12.06,38.23 8.26,35.69 10.16,35.69 9.53,34.04 17.78,40.13 0.64,11.56 0.64,16.64 0.64,14.1 0.64,9.02 0.64,22.35 0.64,24.89 14.86,23.24 16.51,24.26 0.64,36.96 0.64,39.5 0.64,42.04 0.64,44.58 0.64,47.12 0.64,50.29 3.17,51.56 6.35,51.56 9.53,51.56 12.06,50.29 15.75,45.97 17.27,45.97 17.78,48.39 12.45,26.8 10.29,26.16 8.76,25.53 13.97,28.07 17.78,25.53 16.51,18.54 14.1,16.76 15.11,17.78 13.34,22.73 10.92,21.34 4.45,26.8 4.45,34.42 10.16,2.03 13.34,1.4 24.77,1.4 18.29,43.12 5.84,44.07 7.24,44.07 2.41,47.5 2.41,49.66 5.97,47.5 27.94,38.23 38.73,45.21 42.04,45.21 50.8,45.21 54.23,45.21 33.4,35.18 55.31,40.13 58.99,43.31 59.75,48.39 1.27,32.51 1.27,28.7 2.54,28.7 2.54,32.51
  pour Bottom (isolate 0.254, rank 6): 0,0.13 68.58,0.13 68.58,53.47 0,53.47
  pour Top (isolate 0.254, rank 6): 0,0.13 68.58,0.13 68.58,53.47 0,53.47
N$1
  Top 0.254: U2.7 13.82,37.87 14.1,37.59
  Top 0.61: 14.1,37.59 14.48,37.21 14.48,36.32 15.11,35.69 16.38,35.69 17.02,35.05 17.02,32.77 16.45,32.2 14.92,32.2 14.22,31.5 R1.2
  Top 0.813: R1.2 R3.2
N$2
  Top 0.203: R10.2 12.45,2.54 RST.+
N$3
  Top 0.203: R9.2 PWR.+
N$4
  Top 0.203: U2.9 13.97,38.87 14.41,39.31 14.48,39.37 14.61,39.5 14.61,43.18 R26.2
N$5  (via drill 0.3 pad 0.64)
  Top 0.203: TX.- 3.17,41.4 5.71,41.4 v5.97,41.66 | U2.14 12.18,41.92 v12.06,42.04
  Bottom 0.203: v5.97,41.66 11.68,41.66 v12.06,42.04
N$7  (via drill 0.3 pad 0.64)
  Top 0.406: J3.1 4.82,31.91 | 4.82,31.91 5.36,31.91 5.59,32.13 | 4.82,31.91 4.82,32 5.84,33.02
  Top 0.61: 6.22,33.4 6.1,33.53 | 6.1,33.66 6.22,33.53 6.86,33.53 | v8.26,33.53 7.11,33.53 6.86,33.53 | 6.86,33.53 6.48,33.91 | 6.86,33.53 6.35,33.02
  Top 0.813: 5.59,32.13 6.1,32.64 6.1,33.02
  Top 1.016: 6.1,33.02 6.1,33.53 6.1,33.66
  Top 1.27: F1.1 2.54,36.58 3.3,35.81 5.21,35.81 6.1,34.93 6.1,33.66 6.1,33.02
  Bottom 0.61: TP1.T v8.26,33.53
N$10  (via drill 0.3 pad 0.64)
  Top 0.203: RX.- 2.41,42.8 3.17,42.04 v4.7,42.04 | U2.13 12.68,41.64 v13.08,42.04
  Bottom 0.203: v13.08,42.04 12.45,42.67 5.33,42.67 v4.7,42.04
N$11  (via drill 0.3 pad 0.64)
  Top 0.203: J3.3 6.99,30.61 | 6.99,30.61 7.81,30.61 v8.26,30.16 | D9.1 6.99,30.61 | R14.1 11.43,32.77 v11.43,32.39
  Bottom 0.203: TP4.T v8.26,30.16 8.26,30.23 8.51,30.48 9.14,30.48 10.03,31.37 10.03,32.89 10.41,33.27 11.43,33.27 11.68,33.02 11.68,32.64 v11.43,32.39
N$13
  Top 0.203: R12.2 L.+
N$17
  Top 0.203: U2.20 8.9,39.87 8.64,40.13 8.64,42.16 R18.1
N$18
  Top 0.203: U2.21 8.77,39.37 8.13,40.01 8.13,43.43 R17.1
N$36
  Top 0.203: R2.1 RX.+
N$37
  Top 0.203: R13.1 TX.+
PB0  (via drill 0.3 pad 0.64)
  Top 0.203: U3.9 38.86,48.13 29.21,48.13 26.8,45.72 26.8,26.92 v27.05,26.67 27.05,24.13 23.37,20.45 15.1,20.45 11.68,17.03 U4.12
  Bottom 0.203: D7.2 32.02,26.8 27.18,26.8 v27.05,26.67
PB1
  Top 0.203: U3.10 36.7,48.51 28.96,48.51 26.42,45.97 26.42,24 23.24,20.83 14.89,20.83 11.18,17.12 U4.13
PB2
  Top 0.203: U3.11 34.54,48.9 28.7,48.9 26.04,46.23 26.04,24.13 23.11,21.21 14.72,21.21 10.68,17.17 U4.14
PB3/MOSI  (via drill 0.3 pad 0.64)
  Top 0.203: U3.12 32.38,49.28 28.45,49.28 25.4,46.23 v25.4,31.88 25.4,24 22.99,21.59 14.57,21.59 10.18,17.2 U4.15
  Bottom 0.203: U3.34 64.77,26.8 62.87,26.8 62.23,27.43 62.23,30.5 60.85,31.88 v25.4,31.88
PB4/MISO  (via drill 0.3 pad 0.64)
  Top 0.203: U4.16 9.68,17.22 14.43,21.97 22.86,21.97 24.77,23.88 v24.77,32.51 24.77,46.23 28.19,49.66 30.23,49.66 U3.13
  Bottom 0.203: v24.77,32.51 61.59,32.51 U3.38
PB5/SCK  (via drill 0.3 pad 0.64)
  Top 0.203: U4.17 9.08,17.19 14.24,22.35 22.73,22.35 24.13,23.75 v24.13,33.15 24.13,46.48 v24.38,46.74 28.57,50.93 U3.14 | R12.1 v6.86,49.28
  Bottom 0.203: U3.37 64.77,29.34 64.77,31.88 63.5,33.15 v24.13,33.15 | v6.86,49.28 9.27,49.28 11.05,47.5 11.18,47.37 11.81,46.74 v24.38,46.74
PC0  (via drill 0.3 pad 0.64)
  Top 0.203: U4.23 8.53,12.85 8.26,12.57 v8.26,10.29
  Bottom 0.203: U3.19 47.37,6.1 38.1,6.1 34.37,9.83 A0.1 23.54,9.83 21.59,7.87 20.19,7.87 18.53,9.54 11.95,9.54 11.21,8.79 9.5,8.79 8.26,10.03 v8.26,10.29
PC1  (via drill 0.3 pad 0.64)
  Top 0.203: U4.24 8.92,12.35 8.89,12.32 v8.89,10.92
  Bottom 0.203: U3.20 49.53,6.48 38.37,6.48 A0.2 31.48,10.29 23.37,10.29 21.46,8.38 20.32,8.38 18.73,9.97 11.75,9.97 10.94,9.16 9.77,9.16 8.89,10.03 v8.89,10.92
PC2  (via drill 0.3 pad 0.64)
  Top 0.203: U4.25 9.68,11.27 9.53,11.11 9.53,10.16 9.91,9.78 v10.29,9.78 | v25.4,11.18 30.1,6.48 52.07,6.48 U3.21
  Bottom 0.203: v25.4,11.18 23.5,11.18 22.15,9.83 A2.1 20.91,9.83 20.29,10.44 11.65,10.44 10.99,9.78 v10.29,9.78
PC3  (via drill 0.3 pad 0.64)
  Top 0.203: U3.22 53.98,7.11 30.86,7.11 v26.16,11.81 | U4.26 10.18,10.69 v10.16,10.67
  Bottom 0.203: v26.16,11.81 20.97,11.81 A2.2 20.05,10.92 11.56,10.92 11.3,10.67 v10.16,10.67
PC4/SDA  (via drill 0.3 pad 0.64)
  Top 0.203: v31.75,8.38 41.64,8.38 I2C..2 | U3.17 22.86,49.4 22.86,24.26 v22.23,23.62 | U4.27 10.68,11.23 10.79,11.11 10.79,10.41 11.05,10.16 R16.2 11.56,8.89 v12.19,8.26
  Bottom 0.203: I2C..2 I2C...2 60.96,8.02 U3.23 | v31.75,8.38 23.11,8.38 21.84,7.11 19.68,7.11 18.29,8.51 13.34,8.51 13.08,8.26 v12.19,8.26 11.94,8 9.14,8 7.24,9.91 7.24,11.37 8.89,13.02 8.89,15.67 13.67,20.45 19.68,20.45 22.23,22.99 v22.23,23.62
PC5/SCL  (via drill 0.3 pad 0.64)
  Top 0.203: U3.24 63.5,3.48 I2C...1 | I2C..1 43.01,7.75 31.11,7.75 30.86,8 v30.86,9.02 | U3.18 22.23,47.5 v22.23,24.89 | U4.28 11.18,10.79 12.83,9.14 v12.83,8.89 12.83,7.9 12.29,7.37 R19.2
  Bottom 0.203: I2C...1 I2C..1 | v30.86,9.02 23.24,9.02 21.72,7.49 19.94,7.49 18.54,8.89 v12.83,8.89 11.94,8.89 11.43,8.38 9.27,8.38 7.62,10.03 7.62,11.18 9.27,12.83 9.27,15.52 13.82,20.07 19.94,20.07 22.86,22.99 22.86,24.26 v22.23,24.89
PD0/RX  (via drill 0.3 pad 0.64)
  Top 0.203: U3.1 63.5,44.12 UART.1 54.94,35.56 35.56,35.56 34.92,34.93 v34.92,34.42 34.92,22.99 33.91,21.97 28.96,21.97 24.38,17.4 20.7,17.4 19.94,16.64 19.94,11.43 18.77,10.26 12.98,10.26 12.18,11.07 U4.30 | v19.05,44.58 19.18,44.45 19.18,37.08 20.32,35.94 v20.32,34.42 | Q1.3 6.48,46.61 R7.1 v9.14,48.51
  Bottom 0.203: v34.92,34.42 v20.32,34.42 | v9.14,48.51 13.08,44.58 v19.05,44.58
PD1/TX  (via drill 0.3 pad 0.64)
  Top 0.203: U3.2 60.96,43.58 UART.2 53.32,35.94 35.18,35.94 34.29,35.05 v34.29,33.78 34.29,23.11 33.66,22.48 28.96,22.48 24.26,17.78 20.32,17.78 19.43,16.89 19.43,11.56 18.54,10.67 13.24,10.67 12.68,11.22 U4.31 | v21.34,33.78 21.34,35.56 19.68,37.21 19.68,44.83 16.76,47.75 Q2.3 13.84,46.99 R8.1
  Bottom 0.203: v34.29,33.78 v21.34,33.78
PD2/INT0
  Top 0.203: 13.18,11.59 U4.32 14.03,11.75 14.73,11.05 18.29,11.05 19.05,11.81 19.05,17.14 20.07,18.16 24.13,18.16 32,26.04 32,34.8 33.53,36.32 43.64,36.32 D2.1 49.7,37.77 58.42,46.48 U3.3
PD3/INT1
  Top 0.203: U4.1 14.07,12.35 14.99,11.43 18.03,11.43 18.67,12.07 18.67,17.42 19.79,18.54 24,18.54 31.62,26.16 31.62,36.37 D3.1 43.09,37.77 D2.2 51.07,39.77 55.88,44.58 U3.4
PD4
  Top 0.203: U3.5 49.02,46.61 32.64,46.61 31.75,45.72 31.75,40.01 | U4.2 14.33,12.85 15.37,11.81 17.78,11.81 18.29,12.32 18.29,17.69 19.52,18.92 23.88,18.92 31.24,26.29 31.24,39.24 31.75,39.75 | 31.75,39.75 31.75,40.01 | D3.2 31.99,39.77 | 31.99,39.77 31.77,39.77 31.75,39.75 | 31.99,39.77 31.75,40.01
  Bottom 0.203: D3.2 22.95,39.77 D4.1
PD5  (via drill 0.3 pad 0.64)
  Top 0.203: U3.6 46.86,46.99 32.38,46.99 31.11,45.72 v31.11,40.51 30.86,40.26 30.86,26.8 v28.96,24.89 28.96,24.51 23.75,19.3 15.64,19.3 13.18,16.85 U4.9 13.14,16.48
  Bottom 0.203: D5.1 55.07,21.72 32.13,21.72 v28.96,24.89 | v31.11,40.51 21.7,40.51 D4.2
PD6  (via drill 0.3 pad 0.64)
  Top 0.203: U3.7 44.7,47.37 32.13,47.37 30.48,45.72 30.48,27.18 28.83,25.53 v28.32,25.53 28.32,24.38 23.62,19.68 15.44,19.68 12.68,16.93 U4.10
  Bottom 0.203: D5.2 55.15,23.8 D6.1 43.64,22.35 32.38,22.35 29.21,25.53 v28.32,25.53
PD7  (via drill 0.3 pad 0.64)
  Top 0.203: U3.8 42.55,47.75 31.88,47.75 30.1,45.97 30.1,27.56 28.7,26.16 v27.69,26.16 27.69,24.26 23.5,20.07 15.25,20.07 12.18,17 U4.11
  Bottom 0.203: D6.2 43.09,23.8 D7.1 32.97,23.8 30.61,26.16 v27.69,26.16
RESET  (via drill 0.3 pad 0.64)
  Top 0.203: U4.29 11.68,10.98 12.75,9.91 13.59,9.91 13.97,9.53 C6.2 R11.2 16.13,8.89 16.89,8.13 v16.89,7.49 16.89,5.84 16.89,5.71 | RESET.2 v21.84,5.46 17.14,5.46 | 17.14,5.46 17.02,5.46 16.89,5.33 | RST.- 14.1,2.54 16.89,5.33 | 16.89,5.71 16.89,5.33 | 16.89,5.71 17.14,5.46
  Bottom 0.203: U3.30 30.23,5.46 v21.84,5.46 | U3.36 57.78,31.24 20.7,31.24 19.81,30.35 19.81,26.29 15.49,21.97 12.92,21.97 6.35,15.4 6.35,9.76 6.37,9.76 8.89,7.24 16.64,7.24 v16.89,7.49
UART_RX
  Top 0.203: R5.1 Q1.2 8,44.83 R17.2
UART_TX
  Top 0.203: Q2.2 10.29,46.86 R6.1 R18.2
USB_D
  Top 0.203: U2.4 11.68,35.69 R15.2
USB_D+
  Top 0.203: U2.3 11.18,34.8 R14.2
VCC  (via drill 0.3 pad 0.64)
  Top 0.254: U2.8 14.36,38.37 14.48,38.48
  Top 0.305: U4.18 7.39,15.35 | U4.6 14.49,14.85 14.73,14.61 v14.73,13.72 14.6,13.85 U4.4 | D1.1 7.37,37.97
  Top 0.406: R10.1 12.32,5.59 12.83,6.1 | 12.83,6.1 v13.21,6.48 | 12.83,6.1 13.59,6.1 | R9.1 26.04,7.87 | 26.04,7.87 26.48,8.32 | 26.04,7.87 26.04,8.76 | 26.04,7.87 26.92,7.87
  Top 0.61: R16.1 R19.1 v7.62,7.37 | C9.2 5.59,15.37 | 5.59,15.37 C7.2 5.71,16 | 7.39,15.35 6.37,15.35 | 6.33,15.35 5.61,15.35 5.59,15.37 | 5.71,16 5.84,16 6.1,16.26 | 6.1,16.26 v6.99,17.14 | 6.37,15.35 5.71,16 | 6.37,15.35 6.33,15.35 | 6.33,15.35 5.71,14.73 | 6.1,16.26 6.1,15.37 | 15.37,38.48 15.75,38.48 | 14.48,38.48 14.73,38.48 | 14.73,38.48 15.37,38.48 | 15.37,38.48 15.62,38.23 | 14.73,38.48 14.73,38.61 15.62,39.5 | R11.1 15.49,6.6 15.11,6.22 13.46,6.22 v13.21,6.48 | 7.37,37.97 v8,37.97 | C21.2 14.22,45.21 R26.1 13.84,45.21 12.32,43.69 R8.2 | R7.2 v8.38,46.23 | 41.78,15.62 41.91,15.62 42.62,14.91 | 41.53,15.62 41.53,15.49 42.16,14.86 | 41.4,14.99 41.4,14.86 40.77,14.22
  Top 0.813: D5.3 58.05,27.8 62.87,22.99 66.67,22.99 67.69,24 67.69,28.96 U3.33 | U3.28 36.2,4.57 30.99,4.57 | 30.99,4.57 30.23,4.57 | U3.31 30.48,4.06 | 30.48,4.06 30.99,4.57 | A2.3 20.97,13.83 26.04,8.76 26.48,8.32 26.92,7.87 30.23,4.57 | 16.64,29.72 C34.2 18.92,29.72 | 16.64,29.72 C33.2 R1.1 | C8.1 15.75,38.48 C10.1 | v15.75,42.8 C21.2 C22.2 | v29.21,42.8 C20.2 C19.2 | v29.21,27.8 C28.1 C27.1 | v51.82,41.78 C15.2 C16.2 | v41.27,41.78 C18.2 C17.2 | v41.27,28.56 C26.1 C25.1 | v41.27,28.56 41.27,28.54 | v41.27,27.8 41.27,28.32 41.27,28.54 | v53.34,27.8 C24.1 C23.1 | v53.34,13.83 C36.2 C35.2 | C37.1 C38.1 41.4,15.62 | C30.1 C29.1 | C29.1 29.96,14.1 v30.23,13.83 | C32.2 C31.2 C29.1 | v8.64,37.34 v8,37.97 7.94,37.97 7.81,37.85 | v16,39.12 15.49,39.12 v15.24,39.12 15.62,39.5 15.75,39.62 | U1.3 8,24.51 8.51,24 | 8.51,24 v8.64,23.88 | 8.51,24 C4.1 11.18,24 11.43,24.26 | 16.64,29.72 17.02,29.34 17.02,28.7 | 41.4,15.62 41.53,15.62 41.78,15.62 42.55,16.38 | 41.27,28.54 v41.26,28.56 v41.27,28.56 | 30.48,4.06 30.48,4.32 30.23,4.57 | 41.4,15.62 41.4,14.99 41.4,13.95 | 41.4,13.95 41.27,13.83 | 42.16,14.86 42.16,14.46 v41.78,14.08 | v41.78,14.08 41.53,14.08 41.4,13.95 | v41.78,14.08 v40.77,14.08 40.77,13.84 41.27,13.34
  Top 1.27: F1.2 5.78,37.59 6.03,37.85 7.81,37.85 | 15.49,39.12 15.75,39.12 18.92,35.94 18.92,30.23 | 18.92,30.23 18.92,29.72 18.92,28.83 | 18.92,28.83 18.92,27.8 | A6.3 18.92,27.8 | 18.92,27.8 17.89,27.8 | 17.89,27.8 18.92,28.83 | 18.92,28.83 19.81,27.94 | C14.+ 11.43,24.26 12.95,24.26 16.49,27.8 | 16.49,27.8 18.92,30.23 | 17.89,27.8 16.49,27.8 | 41.27,28.32 42.8,26.8 42.8,15.1 42.62,14.91 v41.78,14.08 v41.27,13.57
  Bottom 0.305: 41.4,13.83 41.4,13.7 v41.27,13.57
  Bottom 0.61: v6.99,17.14 6.99,17.27 7.37,17.65 7.43,17.59 | v8.38,46.23 10.16,46.23 13.59,42.8 14.99,42.8 | v15.75,42.8 15.3,42.8 | 14.99,42.8 15.62,42.16 | 14.99,42.8 15.3,42.8 | 15.3,42.8 15.62,43.12 | 41.78,28.07 41.89,28.07 v41.91,28.05
  Bottom 0.813: v13.21,6.48 8.51,6.48 v7.62,7.37 5.59,9.4 5.59,15.75 v6.99,17.14 7.43,17.59 9.4,19.56 9.4,23.11 v8.64,23.88 | A2.3 19.56,12.45 16,12.45 v14.73,13.72 | 9.02,36.96 v8,37.97 | 15.75,41.78 15.76,41.77 16.62,41.77 16.78,41.77 | v29.21,27.8 29.57,27.8 29.59,27.81 29.59,27.8 | v51.82,41.78 51.32,41.78 51.31,41.77 | v41.27,41.78 40.91,41.78 40.89,41.77 | 15.75,39.24 15.88,39.24 v16,39.12 | 40.56,27.8 40.56,27.85 v41.27,28.56 41.29,28.56 41.78,28.07
  Bottom 1.27: A6.3 v29.21,27.8 29.59,27.8 D7.3 40.56,27.8 v41.27,27.8 D6.3 v53.34,27.8 D5.3 | UART.3 51.31,41.77 D2.3 40.89,41.77 D3.3 29.21,41.77 | I2C...3 v53.34,13.83 I2C..3 41.4,13.83 A0.3 v30.23,13.83 A2.3 | 9.02,36.96 13.46,36.96 15.75,39.24 15.75,40.89 | 15.75,40.89 15.75,41.78 v15.75,42.8 16.78,41.77 D4.3 28.56,41.77 | 16.62,41.77 15.75,40.89 | 29.21,41.77 28.56,41.77 | v29.21,42.8 29.21,42.42 | 29.21,42.42 29.21,41.77 | 28.56,41.77 29.21,42.42 | 29.21,42.42 29.84,41.78
VIO  (via drill 0.3 pad 0.64)
  Top 0.254: U2.5 12.18,36.46 12.32,36.32 12.57,36.32 12.68,36.43 | U2.6 12.68,36.72 | 12.68,36.72 12.68,36.43 | 12.83,36.32 12.79,36.32 12.68,36.43 | 12.68,36.72 12.95,36.45
  Top 0.406: R2.2 R13.2 6.86,40.51 6.1,39.75 5.46,39.75 v4.95,39.24
  Top 0.61: 12.83,36.32 14.22,34.93 C11.1 v14.99,34.67 C1.1 | R3.1 v11.94,29.72 R4.2 11.05,28.6 9.5,27.05 v5.46,27.05
  Bottom 0.406: 5.46,37.59 5.46,38.23 4.95,38.73 v4.95,39.24
  Bottom 0.61: v11.94,29.72 13.97,31.75 13.97,33.66 v14.99,34.67 | v5.46,27.05 5.46,37.59
XTAL1
  Top 0.305: U4.7 14.75,15.35 15.55,14.55 X2.1
XTAL2
  Top 0.305: U4.8 14.2,15.85 15.3,16.95 X2.3

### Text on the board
bPlace: www.seeedstudio.com | by Seeed Studio | v1.1 12/22/2016 | Seeeduino Lotus
tNames: 13 | 12 | 11 | 10 | 9 | 8 | 7 | 6 | 5 | 4 | 3 | 2 | 1 | 0 | SCL | SDA | GND | ~ | ~ | ~ | ~ | ~ | ~ | AREF | TX | RX | GND | GND | GND | GND | VCC | VCC | VCC | VCC | D5 | D4 | D3 | TX | D4 | D3 | D2 | RX | GND | GND | GND | GND | VCC | VCC | VCC | VCC | D6 | A7 | D8 | D7 | D5 | A6 | D7 | D6 | MISO | VCC | SCK | MOSI | RST | GND | GND | GND | GND | GND | VCC | VCC | VCC | VCC | A3 | A1 | SDA | SDA | A2 | A0 | SCL | SCL | ANALOG IN | ADC6 | IOREF | RST | 3V3 | 5V | GND | GND | NC | 0 | 1 | 2 | 3 | 4 | 5
bPlate: A0 | A2 | A4 | SPI | UART

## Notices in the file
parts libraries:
moudle-new: This work is licensed under the Creative Commons Attribution 4.0 International License.
To view a copy of this license,visit:
http://creativecommons.org/licenses/by-sa/4.0
moudle-new: CC-BY-SA
